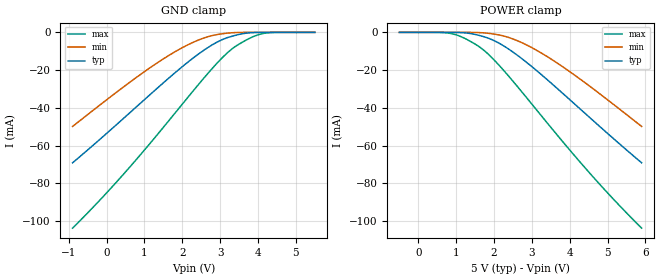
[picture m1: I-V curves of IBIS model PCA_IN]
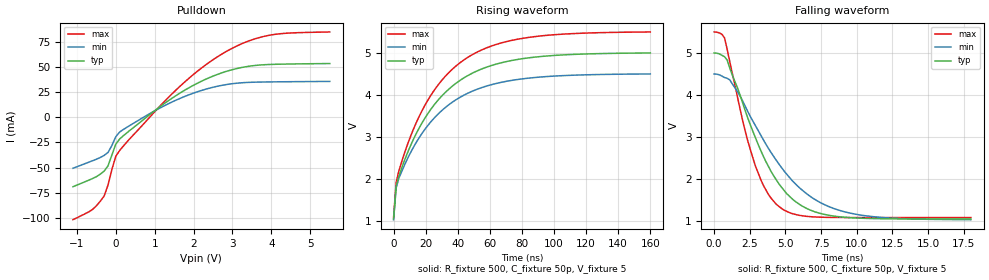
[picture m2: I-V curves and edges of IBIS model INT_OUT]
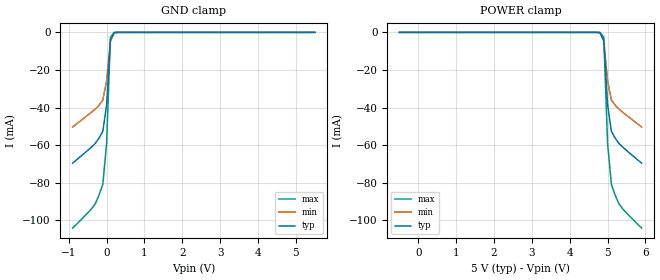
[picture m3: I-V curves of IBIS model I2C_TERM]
|  PCA9541 IBIS MODEL  by NXP Semiconductors, Specialty Logic, Tempe, AZ
|  2-to-1 I2C demultiplexer with interrupt logic and reset
|   Packages: SO16. TSSOP16, HVQFN16
[IBIS Ver]   3.2
[Comment Char]   |_char
| VDD Typ:5V, Min:4.5v, Max: 5.5v
[File name]   pca9541_5v.ibs
[File Rev]   1.0
[Date]   Apr 11, 2008 12:21:34 PM
[Source]
Generated by Seshadri Venkataramanan using IbisToolKit.
[Notes]
[Disclaimer]
(C) Copyright 2007 NXP Semiconductors
All rights reserved
NXP Semiconductors (NXP) does not warrant that this model and any other
accompanying information (Model) accurately or fully represents the
operating characteristics and specifications of the semiconductor
products to which the Model relates.  Moreover, the Model is furnished
on an "as is" and with "all faults" basis, and without support or
warranty of any kind.  NXP disclaims all warranties, whether expressed
or implied or statutory, including without limitation all implied
warranties of non-infringement, merchantability and fitness for any
purpose, and those arising from a course of dealing or usage of trade.
NXP does not convey any license under its or any third party's patents,
copyrights or other intellectual property or proprietary rights.
You and your company assume any and all risks and liability arising out
of the application or use of the Model.
In no event shall NXP be liable for any direct, indirect, special,
consequential or incidental damages, however caused, whether in
warranty, contract or tort (including negligence), strict liability or
other legal theory, including, without limitation, for lost profits,
business interruption, or corruption or loss of data or information,
arising out of or in connection with the use of or the inability to use
the Model, even if NXP has been advised of the possibility of such
damages.
NXP provides the Model as a courtesy to our customers. You and your
company shall not distribute, convey, sell, or give the Model to anyone
else without receiving prior written permission from NXP.
NXP reserves the right to make changes without notice to the Model to
improve reliability, function, or design.
Please be aware that your receipt and subsequent use of the Model shall
serve as acceptance of these terms and conditions.  If you do not
accept these terms, return or destroy the Model immediately.
[Copyright]
2008
[Component]   pca9541-1D
Si_location Pin
Timing_location Pin
[Manufacturer]   NXP Semiconductors
| [Package]   SO16
| [Package]   SO16
[Package]
|  variable   typ   min   max
R_pkg   1.75E-01   1.28E-01   2.11E-01
L_pkg   5.03E-09   3.94E-09   6.26E-09
C_pkg   0.794E-12   0.715E-12   0.869E-12
[Pin] signal_name   model_name   R_pin   L_pin   C_pin
1   INT0B   INT_OUT   1.99E-01  6.26E-09  0.822E-12
2   SDA_MST0   I2C_TERM   2.11E-01  5.46E-09  0.869E-12
3   SCL_MST0   I2C_TERM   1.56E-01  4.44E-09  0.760E-12
4   RESETB   PCA_IN   1.28E-01  3.94E-09  0.717E-12
5   SCL_MST1   I2C_TERM   1.28E-01  3.94E-09  0.715E-12
6   SDA_MST1   I2C_TERM   1.56E-01  4.44E-09  0.760E-12
7   INT1B   INT_OUT   2.11E-01  5.46E-09  0.869E-12
8   VSS   GND   1.99E-01  6.26E-09  0.843E-12
9   A0   PCA_IN   1.99E-01  6.26E-09  0.843E-12
10   A1   PCA_IN   2.11E-01  5.46E-09  0.869E-12
11   A2   PCA_IN   1.56E-01  4.44E-09  0.760E-12
12   A0(I2C_SEL)   PCA_IN   1.28E-01  3.94E-09  0.717E-12
13   SCL_SLAVE   I2C_TERM   1.28E-01  3.94E-09  0.715E-12
14   SDA_SLAVE   I2C_TERM   1.56E-01  4.44E-09  0.760E-12
15   INT_INB   PCA_IN   2.11E-01  5.46E-09  0.869E-12
16   VDD   POWER   1.99E-01  6.26E-09  0.843E-12
[Series Pin Mapping] pin_2 model_name   function_table_group
2   14   PCA_SW1   1
6   14   PCA_SW1   2
3   13   PCA_SW1   1
5   13   PCA_SW1   2
[Series Switch Groups]
|  1 /
On 1 /
|  2/
On 2 /
[Component]   pca9541-1PW
Si_location Pin
Timing_location Pin
[Manufacturer]   NXP Semiconductors
| [Package]   TSSOP16
| [Package]   TSSOP16
[Package]
| variable   typ   min   max
R_pkg   3.95E-02   3.52E-02   4.56E-02
L_pkg   1.94E-09   1.65E-09   2.40E-09
C_pkg   0.446E-12   0.335E-12   0.771E-12
[Pin] signal_name   model_name   R_pin   L_pin   C_pin
1   INT0B   INT_OUT   3.52E-02  2.40E-09  0.436E-12
2   SDA_MST0   I2C_TERM   3.70E-02  1.93E-09  0.438E-12
3   SCL_MST0   I2C_TERM   4.56E-02  1.76E-09  0.345E-12
4   RESETB   PCA_IN   4.00E-02  1.65E-09  0.335E-12
5   SCL_MST1   I2C_TERM   4.00E-02  1.65E-09  0.335E-12
6   SDA_MST1   I2C_TERM   4.56E-02  1.76E-09  0.345E-12
7   INT1B   INT_OUT   3.70E-02  1.93E-09  0.438E-12
8   VSS   GND   3.52E-02  2.40E-09  0.452E-12
9   A0   PCA_IN   3.52E-02  2.40E-09  0.452E-12
10   A1   PCA_IN   3.70E-02  1.93E-09  0.438E-12
11   A2   PCA_IN   4.56E-02  1.76E-09  0.345E-12
12   A0(I2C_SEL)   PCA_IN   4.00E-02  1.65E-09  0.771E-12
13   SCL_SLAVE   I2C_TERM   4.00E-02  1.65E-09  0.771E-12
14   SDA_SLAVE   I2C_TERM   4.56E-02  1.76E-09  0.345E-12
15   INT_INB   PCA_IN   3.70E-02  1.93E-09  0.438E-12
16   VDD   POWER   3.52E-02  2.40E-09  0.452E-12
[Series Pin Mapping] pin_2 model_name   function_table_group
2   14   PCA_SW1   1
6   14   PCA_SW1   2
3   13   PCA_SW1   1
5   13   PCA_SW1   2
[Series Switch Groups]
|  1 /
On 1 /
|  2/
On 2 /
[Component]   pca9541-1BS
Si_location Pin
Timing_location Pin
[Manufacturer]   NXP Semiconductors
[Package]
|  variable   typ   min   max
R_pkg   403m   325m   479m
L_pkg   112nh   98nh   127nh
C_pkg   0.142p   0.129p   0.157p
[Package Model]   hvqfn16
[Pin] signal_name   model_name
1   SCL_MST0   I2C_TERM
2   RESETB   PCA_IN
3   SCL_MST1   I2C_TERM
4   SDA_MST1   I2C_TERM
5   INT1B   INT_OUT
6   VSS   GND
7   A0   PCA_IN
8   A1   PCA_IN
9   A2   PCA_IN
10   A0(I2C_SEL)   PCA_IN
11   SCL_SLAVE   I2C_TERM
12   SDA_SLAVE   I2C_TERM
13   INT_INB   PCA_IN
14   VDD   POWER
15   INT0B   INT_OUT
16   SDA_MST0   I2C_TERM
[Series Pin Mapping] pin_2 model_name   function_table_group
16   12   PCA_SW1   1
4   12   PCA_SW1   2
1   11   PCA_SW1   1
3   11   PCA_SW1   2
[Series Switch Groups]
|  1 /
On 1 /
|  2/
On 2 /
[Define Package Model]   hvqfn16
[Manufacturer]   Unknown
[OEM]   Unknown
[Description]   none
[Number of Pins]   16
[Pin Numbers]
|   1 =
1
|   2 =
2
|   3 =
3
|   4 =
4
|   5 =
5
|   6 =
6
|   7 =
7
|   8 =
8
|   9 =
9
|   10 =
10
|   11 =
11
|   12 =
12
|   13 =
13
|   14 =
14
|   15 =
15
|   16 =
16
[Model Data]
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[End Model Data]
[End Package Model]
[Model]   PCA_SW1
Model_type Series_switch
C_comp   5.5p   5.3p   5.7p
[Temperature Range] 27   85   -40
[Voltage Range]   5   4.5   5.5
[On]
[R Series]   12   4   24
[L Series]   0   0   0
[C Series]   2p   1p   5p
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[Off]
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| Models and submodels in the file (4): PCA_IN (Input), INT_OUT (Open_drain), I2C_TERM (Terminator), PCA_SW1 (Series_switch)
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[Model]   PCA_IN
Model_type Input
Vinh=4
Vinl=1
C_comp   2.44p   2.2p   2.6p
[Temperature Range] 27   85   -40
[Voltage Range]   5   4.5   5.5
[GND Clamp]
-900mV    -69.11mA   -49.84mA   -103.7mA
400mV     -46.41mA   -29.61mA   -76.18mA
1.2V      -32.04mA   -18.02mA   -57.55mA
1.8V      -21.52mA   -10.36mA   -42.94mA
2.2V      -14.94mA   -6.075mA   -33.12mA
2.6V      -9.042mA   -2.788mA   -23.51mA
3V        -4.346mA   -905.4uA   -14.58mA
3.3V      -2.129mA   -223.8uA   -8.962mA
3.7V      -397.7uA   -5.008uA   -3.935mA
4.1V      -8.131uA   -17.99nA   -745.2uA
4.4V      -72.78nA   -636.6pA   -46.39uA
5.5V      14.33pA    135.2pA    41.33fA
[POWER Clamp]
-500mV    14.33pA    135.2pA    41.33fA
600mV     -72.78nA   -636.6pA   -46.39uA
900mV     -8.131uA   -17.99nA   -745.2uA
1.3V      -397.7uA   -5.008uA   -3.935mA
1.7V      -2.129mA   -223.8uA   -8.962mA
2V        -4.346mA   -905.4uA   -14.58mA
2.4V      -9.042mA   -2.788mA   -23.51mA
2.8V      -14.94mA   -6.075mA   -33.12mA
3.2V      -21.52mA   -10.36mA   -42.94mA
3.8V      -32.04mA   -18.02mA   -57.55mA
4.6V      -46.41mA   -29.61mA   -76.18mA
5.9V      -69.11mA   -49.84mA   -103.7mA
[Model]   INT_OUT
Model_type Open_drain
Vref=5
Vmeas=2.5
Rref=500
Cref=50p
C_comp   2.44p   2.2p   2.6p
[Model Spec]
Vmeas   1.65   1.485   1.815
[Temperature Range] 27   85   -40
[Voltage Range]   5   4.5   5.5
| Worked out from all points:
|   slope of the pulldown table from 0 to 0.75 V, typ, clamps not added: 29.4 ohm
|   falling waveform, R_fixture 500, C_fixture 50p, V_fixture 5: 20-80 % time 3.06ns typ, 4.14ns min, 2.09ns max; typ from 5 V to 1.05 V
|   rising waveform, R_fixture 500, C_fixture 50p, V_fixture 5: 20-80 % time 34.9ns typ, 34.3ns min, 34.8ns max; typ from 1.05 V to 5 V
[Pulldown]
-1.1V     -68.86mA   -50.58mA   -101.5mA
-600mV    -60.82mA   -43.16mA   -91.47mA
-300mV    -53.43mA   -37.83mA   -78.17mA
-200mV    -48.22mA   -34.9mA    -67.26mA
0V        -26.68mA   -19.33mA   -38.7mA
200mV     -18.18mA   -12.03mA   -28.34mA
1.4V      17.66mA    14.27mA    21.44mA
2.3V      37.45mA    27.66mA    51.56mA
3V        47.19mA    33.26mA    68.49mA
3.7V      51.74mA    34.86mA    79.07mA
4.3V      52.64mA    35.15mA    83.02mA
5.5V      53.22mA    35.5mA     84.51mA
[Falling Waveform]
R_fixture=500
C_fixture=50p
V_fixture=5
V_fixture_min=4.5
V_fixture_max=5.5
0s        5V         4.5V       5.5V
727.3ps   4.911V     4.416V     5.359V
1.091ns   4.645V     4.36V      4.8V
2ns       3.811V     3.857V     3.387V
2.909ns   2.969V     3.261V     2.294V
3.818ns   2.292V     2.722V     1.627V
4.727ns   1.802V     2.271V     1.3V
6.545ns   1.289V     1.634V     1.11V
8.909ns   1.098V     1.241V     1.084V
18ns      1.048V     1.032V     1.082V
[Rising Waveform]
R_fixture=500
C_fixture=50p
V_fixture=5
V_fixture_min=4.5
V_fixture_max=5.5
0s        1.048V     1.029V     1.082V
1.616ns   1.828V     1.784V     1.918V
6.465ns   2.405V     2.299V     2.576V
12.93ns   2.986V     2.79V      3.232V
19.39ns   3.437V     3.172V     3.742V
25.86ns   3.788V     3.469V     4.137V
42.02ns   4.359V     3.954V     4.78V
59.8ns    4.683V     4.229V     5.144V
80.81ns   4.863V     4.382V     5.346V
160ns     4.996V     4.496V     5.496V
[Ramp]
R_load=500
dV/dt_r   2.355E+0/1.663E-9   2.349E+0/1.378E-9   2.412E+0/4.900E-10
dV/dt_f   2.372E+0/3.532E-10   2.356E+0/6.908E-10   2.365E+0/3.167E-10
|[End   INT_OUT
| [End   SDAX,SCLX
[Model]   I2C_TERM
Model_type Terminator
C_comp   5.5p   5.3p   5.7p
[Temperature Range] 27   85   -40
[Voltage Range]   5   4.5   5.5
[GND Clamp]
-900mV    -69.6mA    -50.37mA   -104.1mA
-400mV    -61.03mA   -42.49mA   -93.95mA
-300mV    -59.07mA   -40.83mA   -91.17mA
-200mV    -56.25mA   -38.7mA    -86.6mA
-100mV    -52.65mA   -35.99mA   -80.77mA
0V        -38.53mA   -26.02mA   -58.95mA
100mV     -4.3mA     -4.638mA   -2.576mA
200mV     -117.7uA   -256.8uA   -20.35uA
5.5V      374.6pA    422pA      378.4pA
[POWER Clamp]
-500mV    374.6pA    422pA      378.4pA
4.8V      -117.7uA   -256.8uA   -20.35uA
4.9V      -4.3mA     -4.638mA   -2.576mA
5V        -38.53mA   -26.02mA   -58.95mA
5.1V      -52.65mA   -35.99mA   -80.77mA
5.2V      -56.25mA   -38.7mA    -86.6mA
5.3V      -59.07mA   -40.83mA   -91.17mA
5.4V      -61.03mA   -42.49mA   -93.95mA
5.9V      -69.6mA    -50.37mA   -104.1mA
